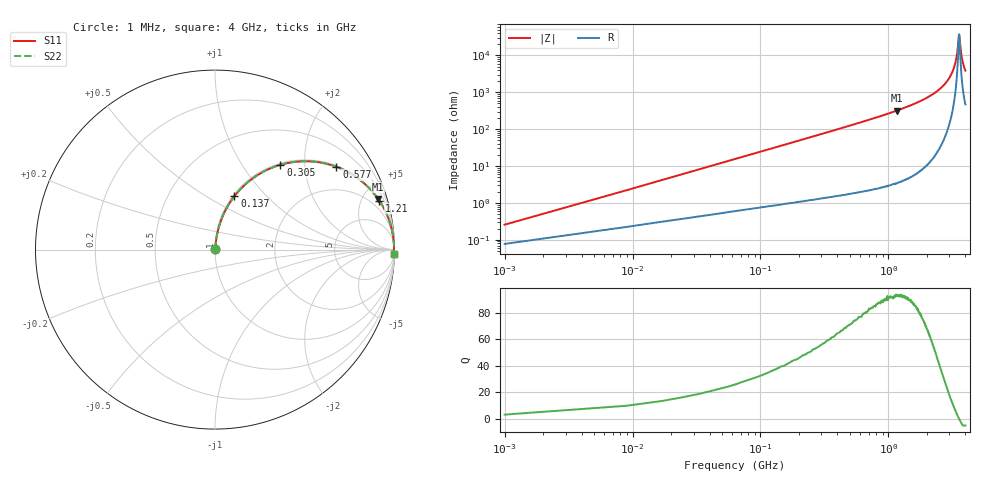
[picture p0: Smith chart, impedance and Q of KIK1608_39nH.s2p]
!version-2
!date-01.2022
!Series
# MHz S RI R 50
!Freq ReS11 ImS11 ReS21 ImS21 ReS12 ImS12 ReS22 ImS22
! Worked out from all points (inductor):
!   501 points, 1 MHz to 4 GHz, reference 50 ohm
!   read as one part in series: L = 39 nH near 17 MHz
!   highest Q = 93.1 at 1.17 GHz (marker M1), where L = 43.6 nH
!   self-resonance near 3.57 GHz
!   S11 on the Smith chart (normalised r, x): 1 MHz: 1.00, +0.00; 137 MHz: 1.02, +0.67; 305 MHz: 1.03, +1.51; 577 MHz: 1.04, +2.90; 1.21 GHz: 1.07, +6.69; 4 GHz: 11, -77
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1  0.000758 0.00245  0.9992 -0.00245  0.9992 -0.00245  0.000758 0.00245
25  0.00744 0.0606  0.9926 -0.0606  0.9926 -0.0606  0.00744 0.0606
41  0.0146 0.0985  0.9854 -0.0985  0.9854 -0.0985  0.0146 0.0985
81  0.0439 0.1886  0.9561 -0.1886  0.9561 -0.1886  0.0439 0.1886
137  0.1078 0.2973  0.8922 -0.2973  0.8922 -0.2973  0.1078 0.2973
305  0.3641 0.4724  0.6359 -0.4724  0.6359 -0.4724  0.3641 0.4724
577  0.6761 0.4614  0.3239 -0.4614  0.3239 -0.4614  0.6761 0.4614
673  0.7425 0.4311  0.2575 -0.4311  0.2575 -0.4311  0.7425 0.4311
1170  0.9089 0.2824  0.0911 -0.2824  0.0911 -0.2824  0.9089 0.2824
1210  0.9155 0.2728  0.0845 -0.2728  0.0845 -0.2728  0.9155 0.2728
1335  0.9332 0.2443  0.0668 -0.2443  0.0668 -0.2443  0.9332 0.2443
2010  0.9791 0.1358  0.0209 -0.1358  0.0209 -0.1358  0.9791 0.1358
2670  0.9934 0.0668  0.00657 -0.0668  0.00657 -0.0668  0.9934 0.0668
3090  0.9966 0.0333  0.00342 -0.0333  0.00342 -0.0333  0.9966 0.0333
3335  0.9973 0.0157  0.00273 -0.0157  0.00273 -0.0157  0.9973 0.0157
3450  0.9974 0.00822  0.00264 -0.00822  0.00264 -0.00822  0.9974 0.00822
3540  0.9973 0.00199  0.00266 -0.00199  0.00266 -0.00199  0.9973 0.00199
3575  0.9973 -4.93e-05  0.00269 4.93e-05  0.00269 4.93e-05  0.9973 -4.93e-05
3660  0.9972 -0.00556  0.00281 0.00556  0.00281 0.00556  0.9972 -0.00556
3740  0.997 -0.0105  0.00296 0.0105  0.00296 0.0105  0.997 -0.0105
3860  0.9967 -0.0176  0.00329 0.0176  0.00329 0.0176  0.9967 -0.0176
4000  0.9962 -0.0254  0.00377 0.0254  0.00377 0.0254  0.9962 -0.0254
